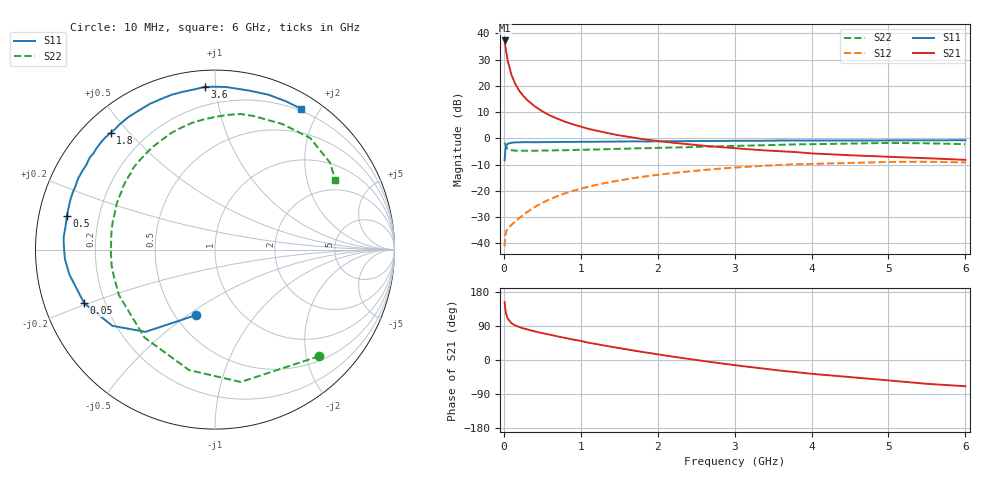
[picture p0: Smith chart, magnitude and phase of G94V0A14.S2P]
! SIEMENS Small Signal Semiconductors
! BFG235
! Si NPN RF Bipolar Junction Transistor in SOT223
! VCE = 4 V  IC = 140 mA
! Common Emitter S-Parameters:  July  1994
# GHz  S  MA  R  50
!  f  S11  S21  S12  S22
! GHz  MAG  ANG  MAG  ANG  MAG  ANG  MAG  ANG
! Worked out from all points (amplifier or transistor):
!   40 points, 10 MHz to 6 GHz, reference 50 ohm
!   highest |S21| = 37.3 dB at 10 MHz (marker M1)
!   |S21| within 3 dB of that: start of sweep to 24.54 MHz
!   unconditionally stable (mu >= 1): 454.2 MHz to 1.485 GHz
!   at 200 MHz: K = 0.81, MSG = 24.3 dB, |S12| = -30.4 dB
!   at 1.5 GHz: K = 1.00, MSG = 8.6 dB, |S12| = -16.0 dB
!   at 6 GHz: K = 0.90, MSG = 0.5 dB, |S12| = -9.2 dB
!   S11 on the Smith chart (normalised r, x): 10 MHz: 0.63, -0.54; 50 MHz: 0.12, -0.19; 500 MHz: 0.08, +0.11; 1.8 GHz: 0.08, +0.44; 3.6 GHz: 0.09, +0.94; 6 GHz: 0.17, +1.77
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0.01  0.3803 -106.2  73.36 152.8  0.0088 62.0  0.8309 -45.6
0.02  0.6 -130.2  57.88 133.9  0.0142 48.5  0.7514 -79.0
0.03  0.7123 -143.4  45.59 122.0  0.0169 41.4  0.6868 -102.1
0.05  0.7876 -157.7  30.44 109.4  0.019 34.8  0.628 -128.7
0.1  0.8234 -170.4  16.08 97.1  0.0225 37.5  0.5922 -154.6
0.15  0.8379 -176.4  10.81 91.0  0.0261 43.7  0.5829 -165.4
0.2  0.8399 -179.4  8.086 87.1  0.0301 48.0  0.5826 -171.5
0.25  0.844 177.4  6.518 83.6  0.0344 51.6  0.5803 -175.7
0.3  0.8459 175.4  5.438 81.0  0.039 54.2  0.5805 -179.2
0.4  0.8428 170.8  4.092 75.6  0.049 57.1  0.5804 175.7
0.5  0.846 167.3  3.27 70.9  0.059 58.1  0.5841 171.4
0.7  0.8529 160.6  2.351 62.1  0.0796 57.7  0.5916 164.1
0.9  0.8544 155.3  1.847 53.9  0.0997 54.8  0.5987 157.8
1.1  0.8591 148.9  1.516 45.7  0.1195 51.3  0.6091 151.6
1.4  0.8643 141.6  1.217 34.8  0.1482 45.4  0.6252 143.1
1.8  0.8726 131.8  0.971 21.3  0.1845 36.7  0.6484 132.1
2.2  0.8821 123.0  0.824 8.7  0.2177 27.7  0.6691 121.4
3.2  0.8973 101.6  0.617 -18.5  0.2893 4.4  0.727 95.4
3.6  0.9084 93.5  0.567 -28.1  0.3111 -5.4  0.754 84.5
4.5  0.906 77.9  0.476 -45.1  0.3391 -25.2  0.7937 61.9
5.5  0.9158 64.7  0.418 -62.9  0.3571 -46.9  0.8033 37.1
6  0.9197 58.5  0.389 -69.2  0.3476 -54.9  0.7746 30.1
